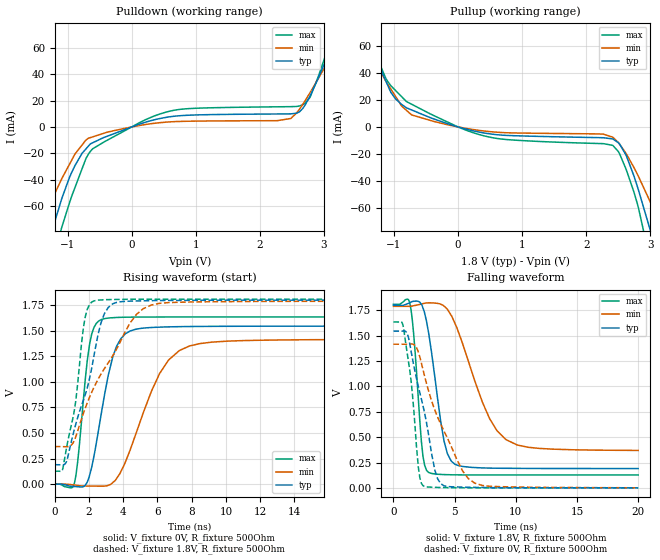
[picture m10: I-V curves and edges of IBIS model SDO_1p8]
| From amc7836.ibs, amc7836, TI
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|   Model
[Model]   SDO_1p8
Model_type   Output
Polarity   Non-Inverting
Vmeas = 0.9
Vref = 0
Cref = 1pF
Rref = 100000
|   typ   min   max
C_comp   2.780pF   2.357pF   3.166pF
[Voltage Range]   1.8   1.79   1.81
[Temperature Range]   27   125   -40
[Pullup Reference]   1.8   1.79   1.81
[Pulldown Reference]   0   0   0
[Power Clamp Reference]   1.8   1.79   1.81
[GND Clamp Reference]   0   0   0
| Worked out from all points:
|   slope of the pulldown table from 0 to 0.27 V, typ, clamps not added: 62.1 ohm
|   slope of the pullup table from 0 to 0.27 V, typ, clamps not added: 83.3 ohm
|   falling waveform, V_fixture 1.8V, R_fixture 500Ohm: 20-80 % time 1.12ns typ, 2.6ns min, 596ps max; typ from 1.8 V to 0.19 V
|   rising waveform, V_fixture 0V, R_fixture 500Ohm: 20-80 % time 1.05ns typ, 2.04ns min, 579ps max; typ from 0 V to 1.55 V
|   rising waveform, V_fixture 1.8V, R_fixture 500Ohm: 20-80 % time 1.44ns typ, 2.57ns min, 817ps max; typ from 0.191 V to 1.8 V
|   falling waveform, V_fixture 0V, R_fixture 500Ohm: 20-80 % time 1.55ns typ, 2.69ns min, 794ps max; typ from 1.54 V to 0 V
[Pulldown]
|   Voltage   I(typ)   I(min)   I(max)
-1.8V     -176.6mA   -119.8mA   -234.2mA
-1.271V   -82.95mA   -57.82mA   -110.5mA
-1.087V   -53.8mA    -38.86mA   -75.48mA
-882mV    -29.02mA   -20.34mA   -45.51mA
-676.8mV  -14.62mA   -8.597mA   -20.72mA
84.6mV    1.513mA    786uA      2.291mA
603mV     7.741mA    3.851mA    12.04mA
2.482V    9.901mA    6.398mA    15.37mA
2.704V    16.5mA     19.76mA    17.88mA
2.785V    23.75mA    26.17mA    22.78mA
2.909V    36.83mA    36.46mA    37.92mA
3.6V      114.8mA    96.34mA    135.9mA
[Pullup]
|   Voltage   I(typ)   I(min)   I(max)
-1.8V     106.2mA    91.41mA    124mA
-1.255V   47.65mA    44.77mA    50.08mA
-1.125V   33.74mA    33.68mA    35.67mA
-974.9mV  20.7mA     22.51mA    26.93mA
-725.4mV  12.58mA    8.913mA    16.81mA
532.8mV   -5.359mA   -3.633mA   -7.934mA
2.412V    -8.894mA   -7.573mA   -13.62mA
2.623V    -21.13mA   -19.87mA   -31.61mA
2.817V    -47.29mA   -37.02mA   -60.74mA
3.044V    -83.98mA   -60.33mA   -109.3mA
3.173V    -106.3mA   -74.68mA   -139.4mA
3.6V      -183.3mA   -125.7mA   -241.3mA
[Ramp]
R_load = 500
|   typ   min   max
dV/dt_r   0.927306/1.04609e-09   0.849611/2.04323e-09   0.981519/5.78852e-10
dV/dt_f   0.965747/1.12486e-09   0.85261/2.6045e-09   1.00988/5.96121e-10
[Falling Waveform]
V_fixture = 1.8V
V_fixture_min = 1.79V
V_fixture_max = 1.81V
R_fixture = 500Ohm
C_fixture = 0F
|   Time   V(typ)   V(min)   V(max)
0s        1.8V       1.79V      1.81V
1.335ns   1.825V     1.79V      1.824V
1.667ns   1.84V      1.796V     1.5V
2.416ns   1.773V     1.817V     310.6mV
2.86ns    1.539V     1.824V     153.4mV
4.14ns    459.1mV    1.792V     130.8mV
5.036ns   231.8mV    1.62V      128.4mV
7.273ns   196.7mV    844.1mV    127.1mV
9.193ns   192.9mV    476.4mV    126.9mV
20ns      190.4mV    369mV      126.9mV
[Rising Waveform]
V_fixture = 0V
V_fixture_min = 0V
V_fixture_max = 0V
R_fixture = 500Ohm
C_fixture = 0F
|   Time   V(typ)   V(min)   V(max)
0s        1.357uV    -7.688uV   238.8nV
1.163ns   -22.97mV   -8.656mV   21.11mV
1.335ns   -24.95mV   -12.81mV   214.2mV
2.035ns   87.56mV    -18.22mV   1.372V
2.708ns   680.8mV    -19.43mV   1.609V
3.387ns   1.244V     15.34mV    1.628V
3.854ns   1.422V     120.6mV    1.632V
6.122ns   1.536V     1.081V     1.635V
7.273ns   1.541V     1.306V     1.636V
20ns      1.546V     1.416V     1.636V
[Rising Waveform]
V_fixture = 1.8V
V_fixture_min = 1.79V
V_fixture_max = 1.81V
R_fixture = 500Ohm
C_fixture = 0F
|   Time   V(typ)   V(min)   V(max)
0s        190.5mV    367.8mV    126.9mV
473.1ps   190.1mV    367.3mV    153.5mV
1.163ns   547.7mV    436.9mV    740.7mV
1.772ns   871.2mV    739.3mV    1.631V
2.281ns   1.249V     944.2mV    1.792V
2.694ns   1.574V     1.075V     1.802V
3.124ns   1.729V     1.187V     1.805V
4.765ns   1.792V     1.659V     1.809V
5.653ns   1.795V     1.753V     1.809V
20ns      1.8V       1.79V      1.81V
[Falling Waveform]
|Gnd
V_fixture = 0V
V_fixture_min = 0V
V_fixture_max = 0V
R_fixture = 500Ohm
C_fixture = 0F
|   Time   V(typ)   V(min)   V(max)
0s        1.545V     1.417V     1.636V
820.5ps   1.547V     1.416V     1.582V
1.444ns   1.349V     1.419V     1.054V
2.035ns   998.9mV    1.339V     203.9mV
2.416ns   809.6mV    1.165V     21.19mV
3.387ns   174.7mV    767.7mV    5.165mV
3.854ns   42.16mV    631.1mV    3.447mV
5.653ns   7.083mV    166.8mV    683.9uV
6.646ns   4.973mV    46.28mV    390.3uV
20ns      -47.76uV   544.8uV    -2.801uV
